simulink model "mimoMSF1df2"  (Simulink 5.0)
settings: Solver=ode45  StartTime=0.0  StopTime=50.0  RelTol=1e-3
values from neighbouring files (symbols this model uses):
  Disturb = Setpoint    [mimo_MSF1DF_sim.m]    (also in mimo_MSF2DF_sim.m)
  K = 1/kpd    [imc2pseucon.m]    (also in imc2pseudo.m)
  Satlb = temp1    [cback.m]    (also in imcmenu.m = str2num(satlbs))
  Satub = temp1    [cback.m]    (also in imcmenu.m = str2num(satubs))
  Setpoint = zeros(1,n)    [mimo_MSF1DF_sim.m]    (also in mimo_MSF2DF_sim.m)
undefined symbols (not defined in the file or in its folder): Ds, input_delay, Kdelay, Ksp, T
libraries: MIMO_lib x8

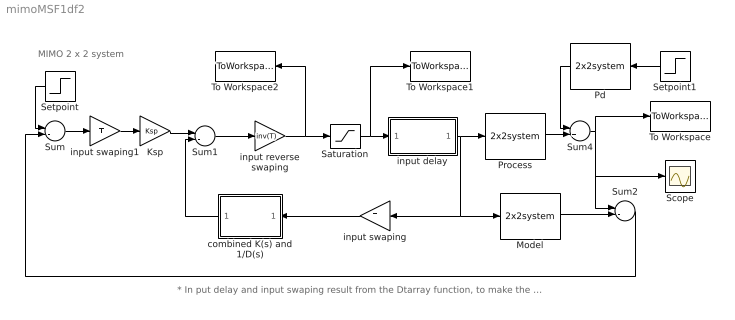
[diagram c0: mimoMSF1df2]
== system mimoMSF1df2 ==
  note: * In put delay and input swaping result from the Dtarray function, to make the system be able to be decoupled.
  note: MIMO 2 x 2 system
  Ksp : Gain  Gain=Ksp  Multiplication=Matrix(K*u)
  Model : MIMO_lib/2x2system  num=Mnum  den=Mden  dead=Mdead
  Pd : MIMO_lib/2x2system  Orientation=left  num=Pdnum  den=Pdden  dead=Pddead
  Process : MIMO_lib/2x2system  num=Pnum  den=Pden  dead=Pdead
  Saturation : Saturate  UpperLimit=Satub  LowerLimit=Satlb
  Scope : Scope
  Setpoint : Step  Orientation=left  Time=0  After=[Setpoint]  SampleTime=0
  Setpoint1 : Step  Orientation=left  Time=0  After=[Disturb]  SampleTime=0
  Sum : Sum  Inputs=+-
  Sum1 : Sum  Inputs=+-
  Sum2 : Sum  Inputs=+-
  Sum4 : Sum
  To Workspace : ToWorkspace  VariableName=yout  SaveFormat=Array
  To Workspace1 : ToWorkspace  VariableName=sat_effort  SaveFormat=Array
  To Workspace2 : ToWorkspace  VariableName=unsat_effort  SaveFormat=Array
  combined K(s) and 1/D(s) : Subsystem  Orientation=left  mask(ksds){Ksp=Ksp, Ds=Ds, Kdelay=Kdelay, K=K}
      mask prompts: Ds "D(s)"; Kdelay "Bdelay"; K "B*(s)"
  input delay : Subsystem  mask(input delay){input_delay=input_delay}
      mask prompts: input_delay "Input Delay (vector)"
  input reverse swaping : Gain  Gain=inv(T)  Multiplication=Matrix(K*u)
  input swaping : Gain  Orientation=left  Gain=T  Multiplication=Matrix(K*u)
  input swaping1 : Gain  Gain=T  Multiplication=Matrix(K*u)
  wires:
  Ksp/1 -> Sum1/1
  combined K(s) and 1/D(s)/1(Out1) -> Sum1/2
  Setpoint/1 -> Sum/1
  input swaping/1 -> combined K(s) and 1/D(s)/1(In1)
  Model/1 -> Sum2/2
  Sum2/1 -> Sum/2
  Process/1 -> Sum4/2
  Sum4/1 -> Sum2/1, To Workspace/1, Scope/1
  input reverse swaping/1 -> Saturation/1, To Workspace2/1
  Sum1/1 -> input reverse swaping/1
  input delay/1(Out1) -> Process/1, Model/1, input swaping/1
  Saturation/1 -> input delay/1(In1), To Workspace1/1
  Setpoint1/1 -> Pd/1
  Pd/1 -> Sum4/1
  input swaping1/1 -> Ksp/1
  Sum/1 -> input swaping1/1

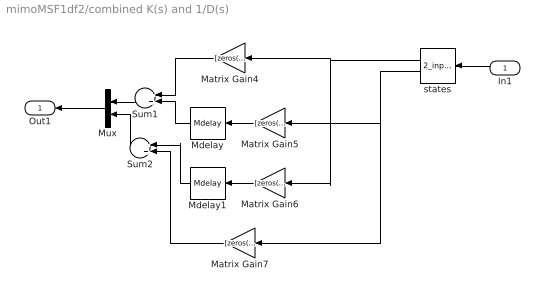
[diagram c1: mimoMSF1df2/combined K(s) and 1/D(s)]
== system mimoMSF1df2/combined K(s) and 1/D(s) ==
  In1 : Inport  Orientation=left
  Matrix Gain4 : Gain  Orientation=left  Gain="[zeros(1,length(Ds{1})-length(K{1,1}))  K{1,1}]"  Multiplication=Matrix(K*u)
  Matrix Gain5 : Gain  Orientation=left  Gain="[zeros(1,length(Ds{2})-length(K{1,2}))  K{1,2}]"  Multiplication=Matrix(K*u)
  Matrix Gain6 : Gain  Orientation=left  Gain="[zeros(1,length(Ds{1})-length(K{2,1}))  K{2,1}]"  Multiplication=Matrix(K*u)
  Matrix Gain7 : Gain  Orientation=left  Gain=[zeros(1,length(Ds{2})-length(K{2,2}) ) K{2,2}]  Multiplication=Matrix(K*u)
  Mdelay : MIMO_lib/Mdelay  Orientation=left  Mdelay=Kdelay(1,2)
  Mdelay1 : MIMO_lib/Mdelay  Orientation=left  Mdelay=Kdelay(2,1)
  Mux : Mux  Orientation=left  Inputs=2
  Sum1 : Sum  Orientation=left
  Sum2 : Sum  Orientation=left
  states : MIMO_lib/2_input_state  Orientation=left  Ds=Ds
  Out1 : Outport  Orientation=left
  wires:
  In1/1 -> states/1
  Sum1/1 -> Mux/1
  Matrix Gain4/1 -> Sum1/1
  Mdelay/1 -> Sum1/2
  Matrix Gain5/1 -> Mdelay/1
  Sum2/1 -> Mux/2
  Matrix Gain6/1 -> Mdelay1/1
  Mdelay1/1 -> Sum2/1
  Matrix Gain7/1 -> Sum2/2
  Mux/1 -> Out1/1
  states/1 -> Matrix Gain4/1, Matrix Gain6/1
  states/2 -> Matrix Gain5/1, Matrix Gain7/1

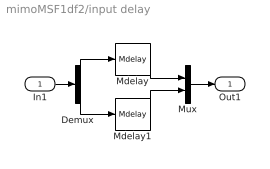
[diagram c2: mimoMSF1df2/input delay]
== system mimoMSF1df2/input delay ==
  In1 : Inport
  Demux : Demux  Outputs=2
  Mdelay : MIMO_lib/Mdelay  Mdelay=input_delay(1)
  Mdelay1 : MIMO_lib/Mdelay  Mdelay=input_delay(2)
  Mux : Mux  Inputs=2
  Out1 : Outport
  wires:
  Mux/1 -> Out1/1
  In1/1 -> Demux/1
  Demux/1 -> Mdelay/1
  Demux/2 -> Mdelay1/1
  Mdelay/1 -> Mux/1
  Mdelay1/1 -> Mux/2
